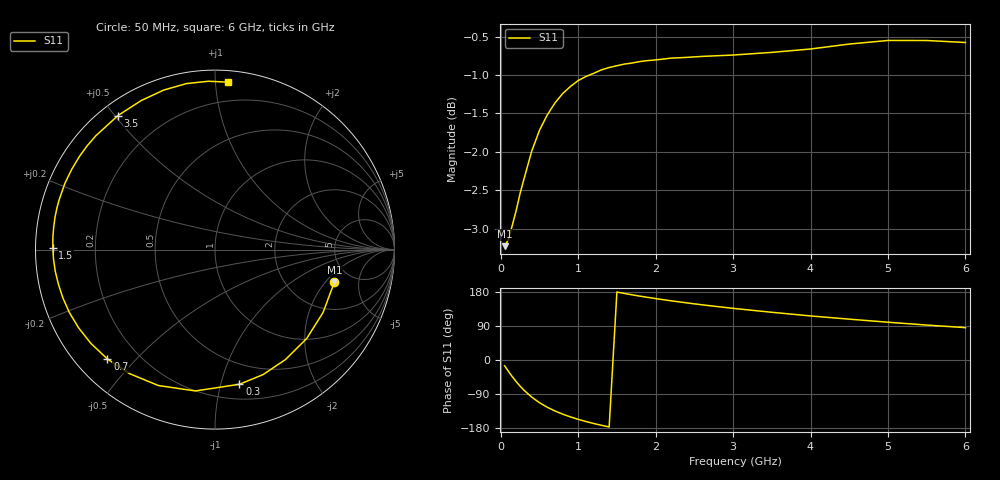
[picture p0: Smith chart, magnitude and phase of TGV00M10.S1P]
! SIEMENS Discrete & RF Semiconductors
! BAT64
! Si Schottky Diode in SOT23
! IF = 0.1 mA
! S-Parameters:  February  1997
# GHz  S  MA  R  50
!  f  S11
! GHz  MAG  ANG
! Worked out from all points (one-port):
!   34 points, 50 MHz to 6 GHz, reference 50 ohm
!   lowest |S11| = -3.2 dB at 50 MHz (marker M1), VSWR 5.44, Z = 181 - j125 ohm
!   |S11| at or under -10 dB: nowhere
!   S11 on the Smith chart (normalised r, x): 50 MHz: 3.61, -2.50; 300 MHz: 0.32, -1.15; 700 MHz: 0.09, -0.42; 1.5 GHz: 0.05, +0.01; 3.5 GHz: 0.05, +0.51; 6 GHz: 0.07, +1.08
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0.05  0.6895 -15.3
0.1  0.6966 -30.2
0.15  0.7116 -44.1
0.2  0.7275 -57.3
0.25  0.7462 -69.0
0.3  0.7626 -79.7
0.4  0.795 -97.9
0.5  0.8203 -112.6
0.6  0.8393 -124.6
0.7  0.8547 -134.5
0.8  0.8668 -142.9
0.9  0.876 -150.2
1  0.8838 -156.6
1.1  0.8893 -162.4
1.3  0.8982 -172.3
1.5  0.9038 179.3
1.6  0.906 175.5
1.8  0.9094 168.4
2  0.9116 162.1
2.4  0.9151 150.8
2.6  0.9165 145.6
3  0.9183 136.3
3.5  0.922 125.9
4  0.9267 116.3
4.5  0.9336 107.8
5  0.9386 99.7
5.5  0.9386 92.2
6  0.9358 85.4
